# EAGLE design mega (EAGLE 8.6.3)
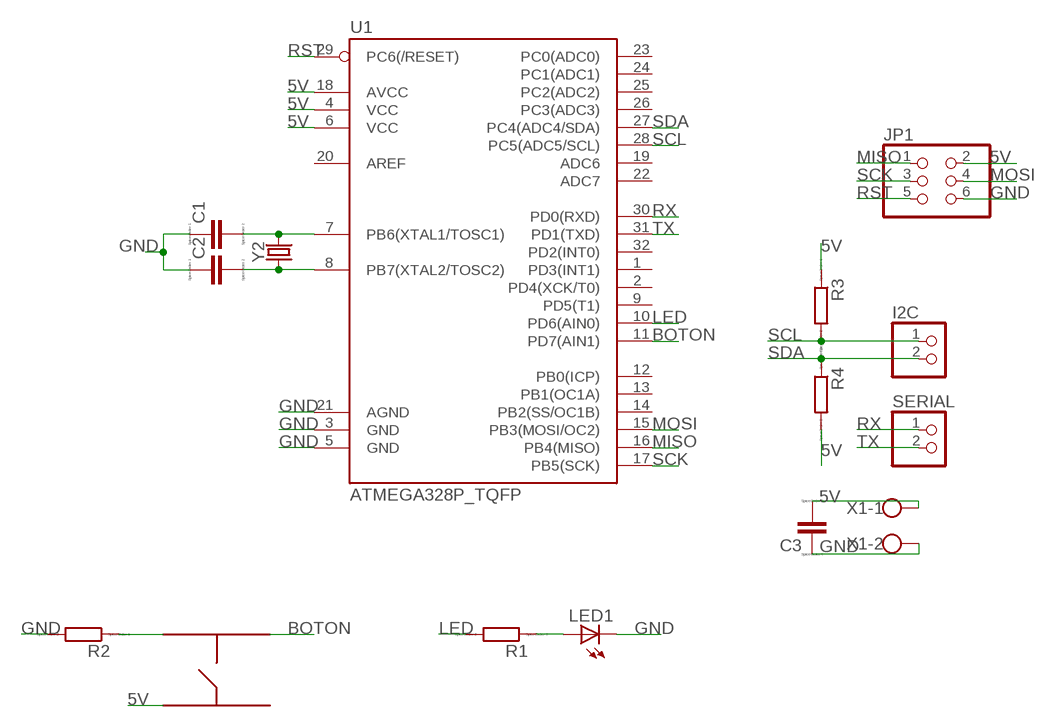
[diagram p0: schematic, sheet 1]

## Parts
C1  CC1206  [C1206]
C2  CC1206  [C1206]
C3  CC1206  [C1206]
I2C  PINHD-1X2  [1X02]
JP1  PINHD-2X3  [2X03]
LED1  LEDSMT1206  [1206]
R1  RR1206  [R1206]
R2  RR1206  [R1206]
R3  RR1206  [R1206]
R4  RR1206  [R1206]
S1  TACTSWITCH  [TACT]
SERIAL  PINHD-1X2  [1X02]
U1  ATMEGA328P_TQFP  [TQFP32-08]
X1  W237-102  [W237-102]
Y2  CRYSTALSMD-HC49UP  [HC49UP]

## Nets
5V: C3.2 JP1.2 R3.1 R4.2 S1.3 U1.4(VCC) U1.6(VCC) U1.18(AVCC) X1.1
BOTON: S1.2 U1.11(PD7(AIN1))
GND: C1.1 C2.1 C3.1 JP1.6 LED1.C R2.2 U1.3(GND) U1.5(GND) U1.21(AGND) X1.2
LED: R1.2 U1.10(PD6(AIN0))
MISO: JP1.1 U1.16(PB4(MISO))
MOSI: JP1.4 U1.15(PB3(MOSI/OC2))
N$1: LED1.A R1.1
N$2: R2.1 S1.1
N$10: C1.2 U1.7(PB6(XTAL1/TOSC1)) Y2.2
N$11: C2.2 U1.8(PB7(XTAL2/TOSC2)) Y2.1
RST: JP1.5 U1.29(PC6(/RESET))
RX: SERIAL.1 U1.30(PD0(RXD))
SCK: JP1.3 U1.17(PB5(SCK))
SCL: I2C.1 R3.2 U1.28(PC5(ADC5/SCL))
SDA: I2C.2 R4.1 U1.27(PC4(ADC4/SDA))
TX: SERIAL.2 U1.31(PD1(TXD))
Unconnected: S1.4 U1.1(PD3(INT1)) U1.2(PD4(XCK/T0)) U1.9(PD5(T1)) U1.12(PB0(ICP)) U1.13(PB1(OC1A)) U1.14(PB2(SS/OC1B)) U1.19(ADC6) U1.20(AREF) U1.22(ADC7) U1.23(PC0(ADC0)) U1.24(PC1(ADC1)) U1.25(PC2(ADC2)) U1.26(PC3(ADC3)) U1.32(PD2(INT0))

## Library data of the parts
C1-C3 = eagle-ltspice:C: CAPACITOR, European symbol; SPICEMODEL: NONE; SPICEPREFIX: C
I2C SERIAL = pinhead:PINHD-1X2: PIN HEADER
JP1 = pinhead:PINHD-2X3: PIN HEADER
LED1 = led:LED: LED
R1-R4 = eagle-ltspice:R: RESISTOR, European symbol; SPICEMODEL: NONE; SPICEPREFIX: R
S1 = oliver:TACTSWITCH
U1 = SparkFun-DigitalIC:ATMEGA328P_TQFP; PROD_ID: IC-09069
X1 = con-wago-500:W237-102: WAGO SCREW CLAMP; MPN: 237-102; OC_FARNELL: unknown; OC_NEWARK: 70K9898
Y2 = SparkFun-Clocks:CRYSTAL: Crystals (Generic)

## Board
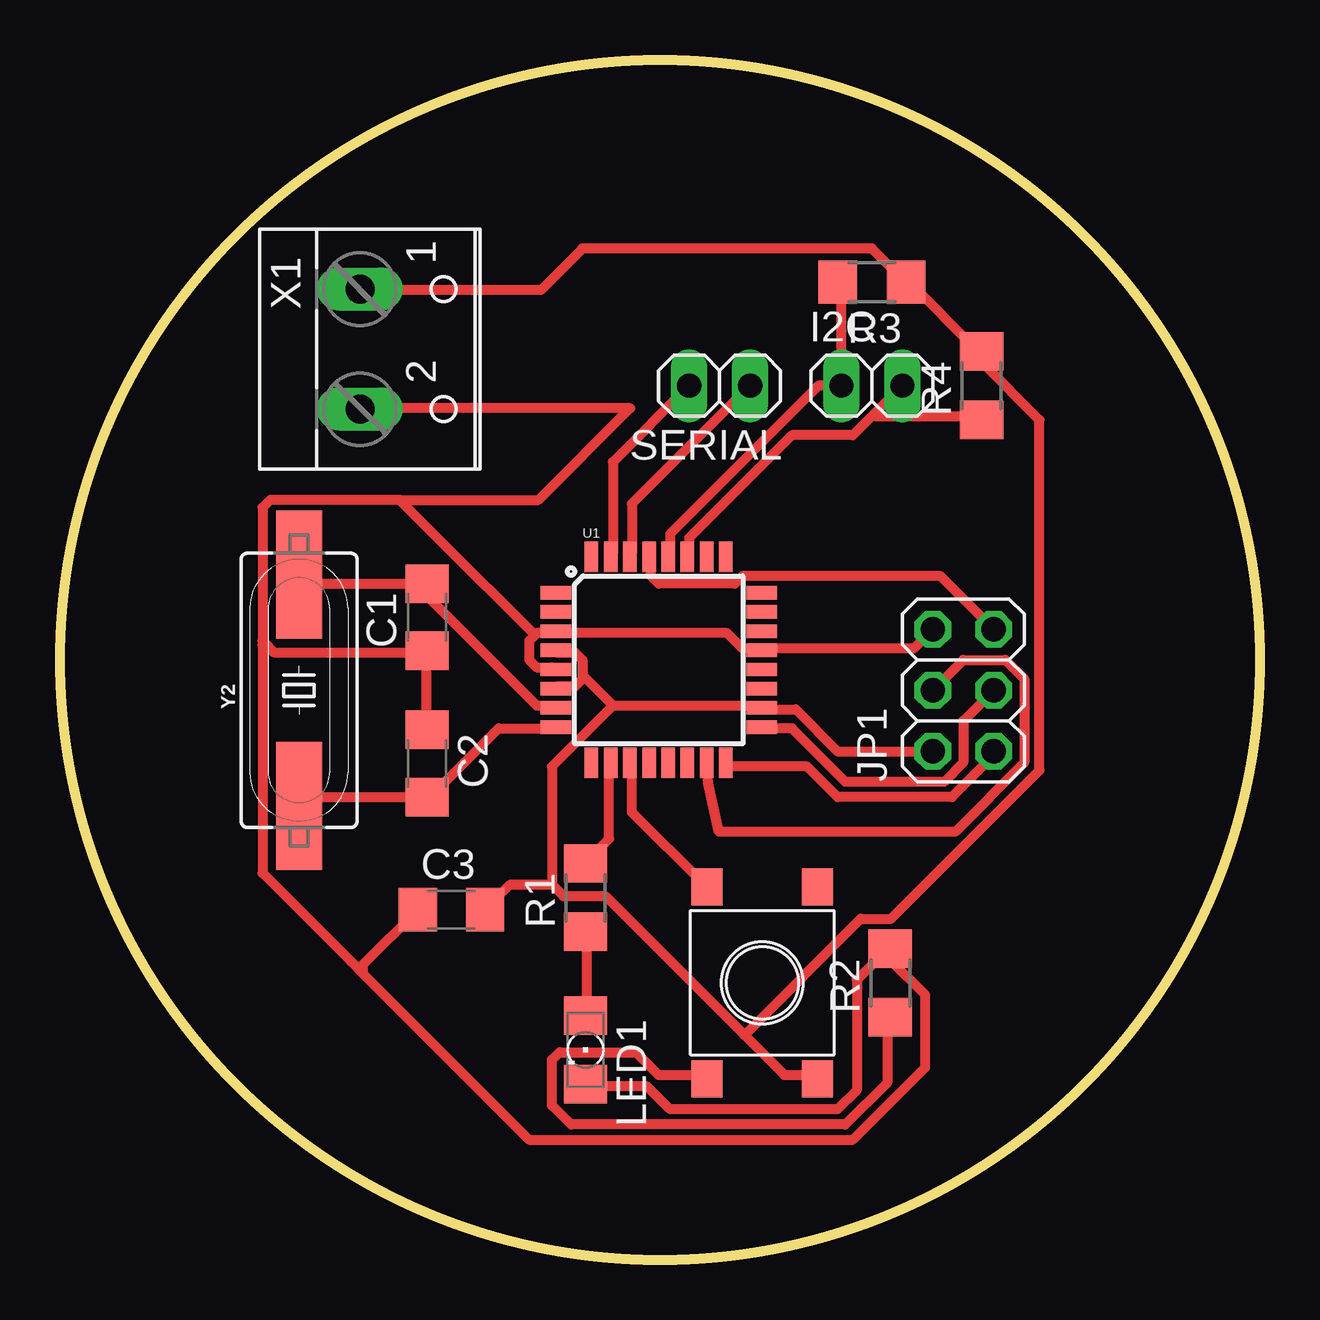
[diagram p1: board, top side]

Size 50.01 x 50.01 mm. Coordinates in mm from the lower left corner, seen from the top.
Outline: circle at 25.01,25.01 radius 25.01
Copper layers (1*16): Top 0.035mm / dielectric 1.5mm / Bottom 0.035mm
Design rules "default *": minimum track width 16mil, minimum drill 0.35mm, track to track 8mil, track to pad 8mil, pad to pad 8mil, via to via 8mil, smd to smd 6mil, copper to edge 40mil, drill to drill 6mil, minimum pad ring 10mil, minimum via ring 8mil, stop-mask expansion 4mil, vias tented up to drill 0mil, thermal gap 10mil

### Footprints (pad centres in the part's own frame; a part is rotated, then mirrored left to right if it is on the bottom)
C1206 = smd 1.6 x 1.8: 1 -1.4,0; 2 1.4,0
1X02 = drill 1.016 long: 1 -1.27,0; 2 1.27,0
2X03 = drill 1.016 octagon: 1 -2.54,-1.27; 2 -2.54,1.27; 3 0,-1.27; 4 0,1.27; 5 2.54,-1.27; 6 2.54,1.27
1206 = smd 1.6 x 1.803: A -1.422,0; C 1.422,0
R1206 = smd 1.6 x 1.803: 1 -1.422,0; 2 1.422,0
TACT = smd 1.55 x 1.3: 1 -4,2.3; 2 4,2.3; 3 -4,-2.3; 4 4,-2.3
TQFP32-08 = smd 1.27 x 0.559: 1 -4.293,2.8; 2 -4.293,2; 3 -4.293,1.2; 4 -4.293,0.4; 5 -4.293,-0.4; 6 -4.293,-1.2; 7 -4.293,-2; 8 -4.293,-2.8; 17 4.293,-2.8; 18 4.293,-2; 19 4.293,-1.2; 20 4.293,-0.4; 21 4.293,0.4; 22 4.293,1.2; 23 4.293,2; 24 4.293,2.8 | smd 0.559 x 1.27: 9 -2.8,-4.293; 10 -2,-4.293; 11 -1.2,-4.293; 12 -0.4,-4.293; 13 0.4,-4.293; 14 1.2,-4.293; 15 2,-4.293; 16 2.8,-4.293; 25 2.8,4.293; 26 2,4.293; 27 1.2,4.293; 28 0.4,4.293; 29 -0.4,4.293; 30 -1.2,4.293; 31 -2,4.293; 32 -2.8,4.293
W237-102 = drill 1.194 long: 1 -2.5,-1.27; 2 2.5,-1.27
HC49UP = smd 5.334 x 1.93: 1 -4.826,0; 2 4.826,0

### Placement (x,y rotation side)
C1  15.3,26.78 90 top
C2  15.3,20.69 270 top
C3  16.32,14.59 0 top
I2C  33.84,36.44 0 top
JP1  37.65,23.74 90 top
LED1  21.91,8.75 270 top
R1  21.91,15.1 90 top
R2  34.61,11.54 90 top
R3  33.84,40.75 180 top
R4  38.42,36.44 90 top
S1  29.27,11.54 90 top
SERIAL  27.49,36.44 180 top
U1  24.95,25.01 0 top
X1  13.78,37.96 270 top
Y2  9.97,23.74 90 top

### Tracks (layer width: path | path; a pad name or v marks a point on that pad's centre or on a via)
5V
  Top 0.406: 21.78,24.21 21.46,23.89 20.67,23.89 U1.6 | 21.78,24.21 21.78,25.01 21.46,25.32 20.67,25.32 U1.4 | 23.05,23.1 29.24,23.1 U1.18 29.4,22.94 30.67,22.94 32.42,21.2 JP1.2 | 23.05,23.1 21.94,24.21 21.78,24.21 | 28.53,9.37 22.73,15.16 20.99,15.16 20.51,15.64 | 28.53,9.37 30.19,7.7 31.46,7.7 S1.3 | 20.51,15.64 20.51,20.56 23.05,23.1 | 28.53,9.37 28.61,9.45 33.37,14.21 34.64,14.21 40.83,20.4 40.83,35.01 38.45,37.39 38.45,37.71 R4.2 38.29,37.86 35.27,40.88 R3.1 35.11,40.88 33.84,42.15 21.78,42.15 20.05,40.42 12.54,40.42 X1.1 | C3.2 18.77,15.64 20.51,15.64
BOTON
  Top 0.406: U1.11 23.84,20.56 23.84,18.66 26.86,15.64 S1.2
GND
  Top 0.406: LED1.C 21.94,7.23 24.48,7.23 25.43,6.27 32.42,6.27 33.21,7.07 33.21,11.67 34.48,12.94 R2.2 34.64,12.78 34.64,12.46 36.07,11.04 36.07,8.02 33.05,5 19.56,5 12.64,11.92 | C2.1 15.27,22.15 15.27,25.32 C1.1 15.11,25.32 8.92,25.32 8.52,25.72 | 19.8,26.04 19.87,26.12 20.51,26.12 U1.3 20.83,26.12 27.81,26.12 28.45,25.48 29.08,25.48 U1.21 29.4,25.48 35.59,25.48 JP1.6 | 19.8,26.04 19.56,25.8 19.56,25.01 19.87,24.69 20.51,24.69 U1.5 | 8.52,25.72 8.44,25.8 8.44,31.36 8.76,31.67 14.16,31.67 | 14.16,31.67 15.91,29.93 19.72,26.12 19.8,26.04 | 12.64,11.92 12.13,12.43 8.44,16.12 8.44,25.64 8.52,25.72 | 12.64,11.92 12.64,12.31 C3.1 | 14.16,31.67 19.94,31.67 23.76,35.5 12.54,35.5 X1.2
LED
  Top 0.406: U1.10 22.89,20.56 22.89,17.54 21.94,16.59 R1.2
MISO
  Top 0.406: JP1.1 38.92,21.04 37.18,19.29 32.42,19.29 31.15,20.56 27.81,20.56 U1.16
MOSI
  Top 0.406: JP1.4 37.65,25.01 39.4,25.01 40.19,24.21 40.19,20.72 37.32,17.84 27.48,17.84 27.02,19.93 27.02,20.56 U1.15
N$1
  Top 0.406: LED1.A 21.94,10.24 21.94,13.58 R1.1
N$2
  Top 0.406: S1.1 26.86,7.7 24.95,7.7 24,8.65 20.83,8.65 20.51,8.34 20.51,6.43 21.3,5.64 32.73,5.64 34.48,7.38 34.48,10.08 R2.1
N$10
  Top 0.406: U1.7 20.51,23.1 19.87,23.1 15.43,27.55 15.43,28.18 C1.2 15.11,28.18 10.35,28.18 10.03,28.5 Y2.2
N$11
  Top 0.406: U1.8 20.51,22.15 18.29,22.15 15.43,19.29 C2.2 15.11,19.29 10.35,19.29 10.03,18.97 Y2.1
RST
  Top 0.406: JP1.5 36.7,28.5 28.45,28.5 28.13,28.18 24.95,28.18 24.64,28.5 24.64,29.29 U1.29
RX
  Top 0.406: SERIAL.1 23.84,31.51 23.84,29.45 U1.30
SCK
  Top 0.406: JP1.3 37.65,22.47 37.65,20.72 36.86,19.93 32.73,19.93 30.51,22.15 29.4,22.15 U1.17
SCL
  Top 0.406: U1.28 25.43,29.45 25.43,30.24 31.62,36.44 I2C.1 32.57,36.59 32.57,40.72 R3.2
SDA
  Top 0.406: I2C.2 33.92,35.24 | 33.92,35.24 33.05,34.37 30.51,34.37 26.22,30.09 26.22,29.45 U1.27 | R4.1 38.29,35.17 34,35.17 33.92,35.24
TX
  Top 0.406: SERIAL.2 23.05,33.26 23.05,29.45 U1.31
